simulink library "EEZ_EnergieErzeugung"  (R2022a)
settings: Solver=VariableStepAuto  StartTime=0.0  StopTime=10.0  RelTol=1e-3
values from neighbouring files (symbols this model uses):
  PAR_EEZ_DCACWirkungsgrad = 0.95    [parameter_EEZ.m]
  PAR_EEZ_Monat = [1, 1, 2, 2, 3, 3, 4, 4, 5, 5, 6, 6, 7, 7, 8, 8, 9, 9, 10, 10, 11, 11, 12, 12]    [parameter_EEZ.m]
  PAR_EEZ_Monate = [1;2;3;4;5;6;7;8;9;10;11;12]    [parameter_EEZ.m]
  PAR_EEZ_Monatstage = [1, 31, 32, 59, 60, 90, 91, 120, 121, 151, 152, 181, 182, 212, 213, 243, 244, 273, 274, 304, 305, 334, 335, 365]    [parameter_EEZ.m]
  PAR_EEZ_NeigungsfaktorS_f64 = [0.9 1 0.7]    [parameter_EEZ.m]
  PAR_EEZ_NeigungsfaktorWO_f64 = [0.9 0.75 0.5]    [parameter_EEZ.m]
  PAR_EEZ_NeigungswinkelS_f64 = [0 45 90]    [parameter_EEZ.m]
  PAR_EEZ_NeigungswinkelWO_f64 = [0 45 90]    [parameter_EEZ.m]
  PAR_EEZ_PVAnzahlModule_O = 0    [parameter_EEZ.m]
  PAR_EEZ_PVAnzahlModule_S = 27    [parameter_EEZ.m]
  PAR_EEZ_PVAnzahlModule_W = 0    [parameter_EEZ.m]
  PAR_EEZ_PVModulbreite_f64 = 0.99    [parameter_EEZ.m]
  PAR_EEZ_PVModullaenge_f64 = 1.68    [parameter_EEZ.m]
  PAR_EEZ_PVNeigungswinkel_O = 45    [parameter_EEZ.m]
  PAR_EEZ_PVNeigungswinkel_S = 45    [parameter_EEZ.m]
  PAR_EEZ_PVNeigungswinkel_W = 45    [parameter_EEZ.m]
  PAR_EEZ_PVWirkungsgrad_f64 = 0.19    [parameter_EEZ.m]
  PAR_EEZ_StrahlungLippstadt = [0 0 0 0 0 0 0 0 0 0 0 0    [parameter_EEZ.m]
  PAR_EEZ_Stunden = [0 1 2 3 4 5 6 7 8 9 10 11 12 13 14 15 16 17 18 19 20 21 22 23]    [parameter_EEZ.m]
  PAR_EEZ_WWKAbsorptionskoeffizient_f64 = 0.94    [parameter_EEZ.m]
  PAR_EEZ_WWKAnzahlModule_f64 = 1    [parameter_EEZ.m]
  PAR_EEZ_WWKModulbreite_f64 = 1.99    [parameter_EEZ.m]
  PAR_EEZ_WWKModullaenge_f64 = 2.455    [parameter_EEZ.m]
  PAR_EEZ_WWKNeigungswinkel_f64 = 45    [parameter_EEZ.m]
  PAR_EEZ_WWKTransmissionskoefffizient_f64 = 0.8    [parameter_EEZ.m]
libraries: embmathops x2

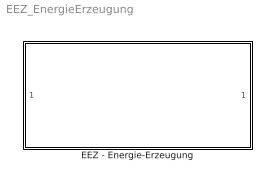
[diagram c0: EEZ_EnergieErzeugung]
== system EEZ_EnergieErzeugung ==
  EEZ - Energie-Erzeugung : Subsystem

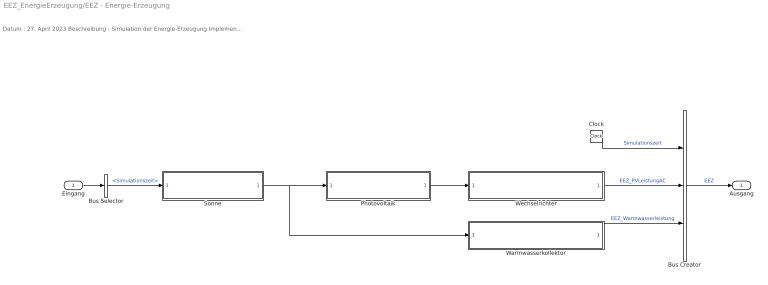
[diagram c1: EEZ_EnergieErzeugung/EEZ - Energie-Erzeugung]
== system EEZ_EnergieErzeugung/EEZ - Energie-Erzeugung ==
  note: Datum : 27. April 2023 Beschreibung : Simulation der Energie-Erzeugung Implementierung : Simulink 10.5 (R2022a) Autor : Daniel Gosedopp & Junjie lyu Bemerkung : Code-Review noch ausstehend Letzte Änderung : 15. Mai 2023
  Eingang : Inport
  Bus Creator : BusCreator  Inputs=3
  Bus Selector : BusSelector  OutputSignals=EEZ.Simulationszeit
  Clock : Clock
  Photovoltaik : Subsystem
  Sonne : Subsystem
  Warmwasserkollektor : Subsystem
  Wechselrichter : Subsystem
  Ausgang : Outport
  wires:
  Bus Selector/1 -> Sonne/1(Eingang)  "<Simulationszeit>"
  Eingang/1 -> Bus Selector/1
  Clock/1 -> Bus Creator/1  "Simulationszeit"
  Wechselrichter/1(EEZ_PVLeistungAC) -> Bus Creator/2  "EEZ_PVLeistungAC"
  Sonne/1(EEZ_Globalstrahlung) -> Warmwasserkollektor/1(EEZ_Globalstrahlung), Photovoltaik/1(Eing_Sonne)
  Bus Creator/1 -> Ausgang/1  "EEZ"
  Warmwasserkollektor/1(EEZ_Warmwasserleistung) -> Bus Creator/3  "EEZ_Warmwasserleistung"
  Photovoltaik/1(EEZ_PVLeistungDC) -> Wechselrichter/1(EEZ_PVLeistungDC)

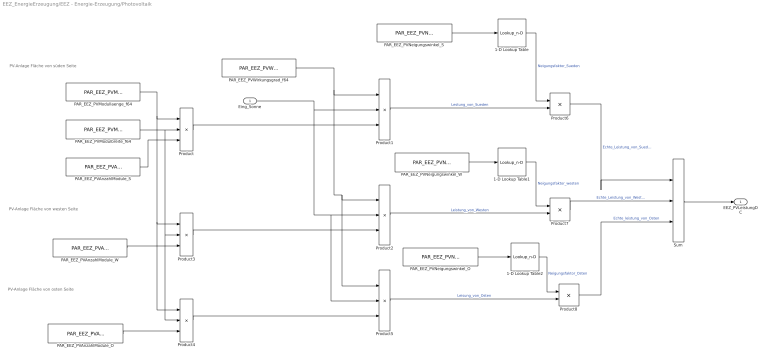
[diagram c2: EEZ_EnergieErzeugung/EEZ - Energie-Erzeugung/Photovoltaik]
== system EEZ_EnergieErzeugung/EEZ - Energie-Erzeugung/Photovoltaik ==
  note: PV-Anlage Fläche von süden Seite
  note: PV-Anlage Fläche von westen Seite
  note: PV-Anlage Fläche von osten Seite
  Eing_Sonne : Inport
  1-D Lookup Table : Lookup_n-D  NumberOfTableDimensions=1  BreakpointsForDimension1=PAR_EEZ_NeigungswinkelS_f64  Table=PAR_EEZ_NeigungsfaktorS_f64  InternalRulePriority=Speed  RndMeth=Simplest
  1-D Lookup Table1 : Lookup_n-D  NumberOfTableDimensions=1  BreakpointsForDimension1=PAR_EEZ_NeigungswinkelWO_f64  Table=PAR_EEZ_NeigungsfaktorWO_f64  InternalRulePriority=Speed  RndMeth=Simplest
  1-D Lookup Table2 : Lookup_n-D  NumberOfTableDimensions=1  BreakpointsForDimension1=PAR_EEZ_NeigungswinkelWO_f64  Table=PAR_EEZ_NeigungsfaktorWO_f64  InternalRulePriority=Speed  RndMeth=Simplest
  PAR_EEZ_PVAnzahlModule_O : Constant  Value=PAR_EEZ_PVAnzahlModule_O
  PAR_EEZ_PVAnzahlModule_S : Constant  Value=PAR_EEZ_PVAnzahlModule_S
  PAR_EEZ_PVAnzahlModule_W : Constant  Value=PAR_EEZ_PVAnzahlModule_W
  PAR_EEZ_PVModulbreite_f64 : Constant  Value=PAR_EEZ_PVModulbreite_f64
  PAR_EEZ_PVModullaenge_f64 : Constant  Value=PAR_EEZ_PVModullaenge_f64
  PAR_EEZ_PVNeigungswinkel_O : Constant  Value=PAR_EEZ_PVNeigungswinkel_O
  PAR_EEZ_PVNeigungswinkel_S : Constant  Value=PAR_EEZ_PVNeigungswinkel_S
  PAR_EEZ_PVNeigungswinkel_W : Constant  Value=PAR_EEZ_PVNeigungswinkel_W
  PAR_EEZ_PVWirkungsgrad_f64 : Constant  Value=PAR_EEZ_PVWirkungsgrad_f64
  Product{,1..5} (6 alike) : Product  Inputs=3
  Product6 : Product
  Product7 : Product
  Product8 : Product
  Sum : Sum  Inputs=|+++
  EEZ_PVLeistungDC : Outport
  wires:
  Product5/1 -> Product8/2  "Leisung_von_Osten"
  Product8/1 -> Sum/3  "Echte_leistung_von_Osten"
  Product7/1 -> Sum/2  "Echte_Leistung_von_Westen"
  Product6/1 -> Sum/1  "Echte_Leistung_von_Sueden"
  1-D Lookup Table2/1 -> Product8/1  "Neigungsfaktor_Osten"
  PAR_EEZ_PVNeigungswinkel_O/1 -> 1-D Lookup Table2/1
  1-D Lookup Table1/1 -> Product7/1  "Neigungsfaktor_westen"
  PAR_EEZ_PVNeigungswinkel_W/1 -> 1-D Lookup Table1/1
  1-D Lookup Table/1 -> Product6/1  "Neigungsfaktor_Sueden"
  PAR_EEZ_PVNeigungswinkel_S/1 -> 1-D Lookup Table/1
  Product2/1 -> Product7/2  "Leistung_von_Westen"
  Product1/1 -> Product6/2  "Lestung_von_Sueden"
  Product4/1 -> Product5/3
  Product3/1 -> Product2/3
  Product/1 -> Product1/3
  Eing_Sonne/1 -> Product1/2, Product5/2, Product2/2
  PAR_EEZ_PVWirkungsgrad_f64/1 -> Product1/1, Product2/1, Product5/1
  PAR_EEZ_PVAnzahlModule_O/1 -> Product4/3
  PAR_EEZ_PVAnzahlModule_W/1 -> Product3/3
  PAR_EEZ_PVAnzahlModule_S/1 -> Product/3
  PAR_EEZ_PVModulbreite_f64/1 -> Product3/2, Product4/2, Product/2
  PAR_EEZ_PVModullaenge_f64/1 -> Product3/1, Product4/1, Product/1
  Sum/1 -> EEZ_PVLeistungDC/1

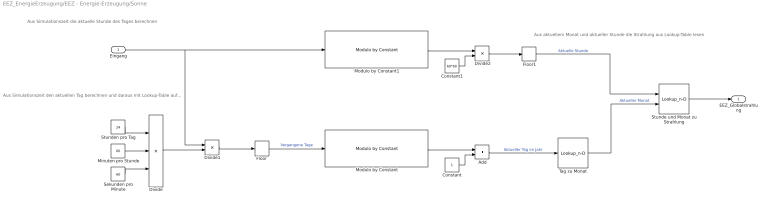
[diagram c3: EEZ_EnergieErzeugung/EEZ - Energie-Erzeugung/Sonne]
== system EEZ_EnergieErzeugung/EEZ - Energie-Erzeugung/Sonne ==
  note: Aus aktuellem Monat und aktueller Stunde die Strahlung aus Lookup-Table lesen
  note: Aus Simulationszeit die aktuelle Stunde des Tages berechnen
  note: Aus Simulationszeit den aktuellen Tag berechnen und daraus mit Lookup-Table auf den aktuellen Monat schließen
  Eingang : Inport
  Add : Sum
  Constant : Constant
  Constant1 : Constant  Value=60*60
  Divide : Product  Inputs=***
  Divide1 : Product  Inputs=*/
  Divide2 : Product  Inputs=*/
  Floor : Rounding
  Floor1 : Rounding
  Minuten pro Stunde : Constant  Value=60
  Modulo by Constant : embmathops/Modulo by Constant  Denominator=365  SimulateUsing=Code generation
  Modulo by Constant1 : embmathops/Modulo by Constant  Denominator=24*60*60  SimulateUsing=Code generation
  Sekunden pro Minute : Constant  Value=60
  Stunde und Monat zu Strahlung : Lookup_n-D  BreakpointsForDimension1=PAR_EEZ_Stunden  BreakpointsForDimension2=PAR_EEZ_Monate  Table=PAR_EEZ_StrahlungLippstadt  InternalRulePriority=Speed  RndMeth=Simplest
  Stunden pro Tag : Constant  Value=24
  Tag zu Monat : Lookup_n-D  NumberOfTableDimensions=1  BreakpointsForDimension1=PAR_EEZ_Monatstage  Table=PAR_EEZ_Monat  InternalRulePriority=Speed  RndMeth=Simplest
  EEZ_Globalstrahlung : Outport
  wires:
  Stunden pro Tag/1 -> Divide/1
  Minuten pro Stunde/1 -> Divide/2
  Sekunden pro Minute/1 -> Divide/3
  Divide/1 -> Divide1/2
  Eingang/1 -> Modulo by Constant1/1, Divide1/1
  Divide1/1 -> Floor/1
  Floor/1 -> Modulo by Constant/1  "Vergangene Tage"
  Modulo by Constant/1 -> Add/1
  Constant/1 -> Add/2
  Add/1 -> Tag zu Monat/1  "Aktueller Tag im Jahr"
  Modulo by Constant1/1 -> Divide2/1
  Constant1/1 -> Divide2/2
  Divide2/1 -> Floor1/1
  Floor1/1 -> Stunde und Monat zu Strahlung/1  "Aktuelle Stunde"
  Stunde und Monat zu Strahlung/1 -> EEZ_Globalstrahlung/1
  Tag zu Monat/1 -> Stunde und Monat zu Strahlung/2  "Aktueller Monat"

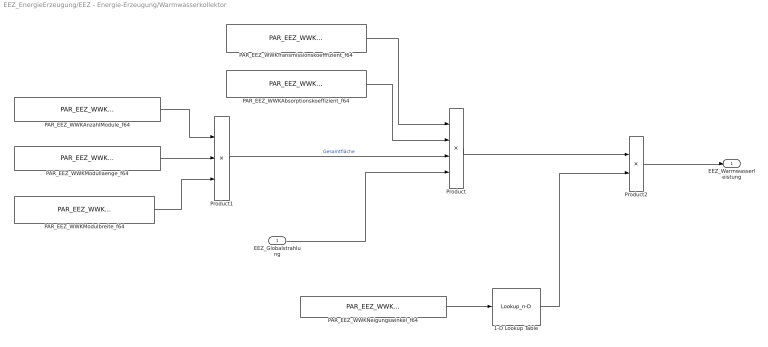
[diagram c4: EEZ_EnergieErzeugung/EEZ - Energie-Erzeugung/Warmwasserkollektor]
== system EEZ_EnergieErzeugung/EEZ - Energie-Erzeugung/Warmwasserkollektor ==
  EEZ_Globalstrahlung : Inport
  1-D Lookup Table : Lookup_n-D  NumberOfTableDimensions=1  BreakpointsForDimension1=PAR_EEZ_NeigungswinkelS_f64  Table=PAR_EEZ_NeigungsfaktorS_f64  InternalRulePriority=Speed  RndMeth=Simplest
  PAR_EEZ_WWKAbsorptionskoeffizient_f64 : Constant  Value=PAR_EEZ_WWKAbsorptionskoeffizient_f64
  PAR_EEZ_WWKAnzahlModule_f64 : Constant  Value=PAR_EEZ_WWKAnzahlModule_f64
  PAR_EEZ_WWKModulbreite_f64 : Constant  Value=PAR_EEZ_WWKModulbreite_f64
  PAR_EEZ_WWKModullaenge_f64 : Constant  Value=PAR_EEZ_WWKModullaenge_f64
  PAR_EEZ_WWKNeigungswinkel_f64 : Constant  Value=PAR_EEZ_WWKNeigungswinkel_f64
  PAR_EEZ_WWKTransmissionskoefffizient_f64 : Constant  Value=PAR_EEZ_WWKTransmissionskoefffizient_f64
  Product : Product  Inputs=4
  Product1 : Product  Inputs=3
  Product2 : Product
  EEZ_Warmwasserleistung : Outport
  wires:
  Product2/1 -> EEZ_Warmwasserleistung/1
  1-D Lookup Table/1 -> Product2/2
  Product/1 -> Product2/1
  PAR_EEZ_WWKNeigungswinkel_f64/1 -> 1-D Lookup Table/1
  EEZ_Globalstrahlung/1 -> Product/4
  PAR_EEZ_WWKAbsorptionskoeffizient_f64/1 -> Product/2
  PAR_EEZ_WWKTransmissionskoefffizient_f64/1 -> Product/1
  Product1/1 -> Product/3  "Gesamtfläche"
  PAR_EEZ_WWKModulbreite_f64/1 -> Product1/3
  PAR_EEZ_WWKModullaenge_f64/1 -> Product1/2
  PAR_EEZ_WWKAnzahlModule_f64/1 -> Product1/1

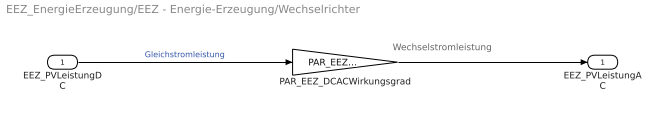
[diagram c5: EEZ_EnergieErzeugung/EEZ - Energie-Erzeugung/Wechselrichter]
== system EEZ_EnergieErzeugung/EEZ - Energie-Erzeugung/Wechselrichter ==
  note: Wechselstromleistung
  EEZ_PVLeistungDC : Inport
  PAR_EEZ_DCACWirkungsgrad : Gain  Gain=PAR_EEZ_DCACWirkungsgrad
  EEZ_PVLeistungAC : Outport
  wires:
  PAR_EEZ_DCACWirkungsgrad/1 -> EEZ_PVLeistungAC/1
  EEZ_PVLeistungDC/1 -> PAR_EEZ_DCACWirkungsgrad/1  "Gleichstromleistung"
